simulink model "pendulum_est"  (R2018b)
settings: Solver=ode4  StartTime=0.0  StopTime=T  FixedStep=1e-3  RelTol=1e-3
model workspace (MAT data in the model file):
  pendulum_down1 : sldodialogs.data.SessionData (value not decoded)
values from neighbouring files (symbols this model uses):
  dtheta0 = mean(dtheta(n_start-5:n_start+5))    [mainSkript_odhadKyvadlaZvlast.m]    (also in mainSkript_pocitaniTVLQR_simplified.m = traj.dth_0; mainSkript_provedeniSimulaceSwingUp.m = [dtheta0 , stbVc])
  k_1 = params.k_1    [mainSkript_odhadKyvadlaZvlast.m]    (also in mainSkript_estimaceVozik.m = 1 / m; mainSkript_kyvadlaNajednouOdhad.m; mainSkript_modifikaceVozik.m = 0.695894224078)
  k_2 = params.k_2    [mainSkript_odhadKyvadlaZvlast.m]    (also in mainSkript_kyvadlaNajednouOdhad.m)
  theta0 = theta_cut(1)    [mainSkript_odhadKyvadlaZvlast.m]    (also in mainSkript_pocitaniTVLQR_simplified.m = traj.th_0; mainSkript_provedeniSimulaceSwingUp.m = [theta0 , stbVc])

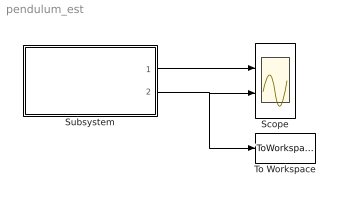
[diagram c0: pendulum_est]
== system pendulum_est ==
  Scope : Scope  NumInputPorts=2
  Subsystem : Subsystem
  To Workspace : ToWorkspace  VariableName=th_sim  SaveFormat=Structure With Time  SampleTime=-1
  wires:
  Subsystem/1(dtheta) -> Scope/1
  Subsystem/2(theta) -> To Workspace/1, Scope/2

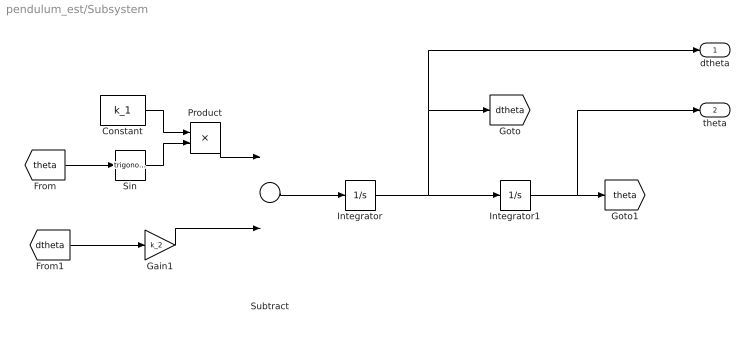
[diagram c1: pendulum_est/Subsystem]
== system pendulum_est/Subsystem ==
  Constant : Constant  Value=k_1
  Gain1 : Gain  Gain=k_2
  Integrator : Integrator  InitialCondition=dtheta0
  Integrator1 : Integrator  InitialCondition=theta0
  Product : Product
  Sin : Trigonometry
  Subtract : Sum  Inputs=+-
  dtheta : Outport
  theta : Outport  Port=2
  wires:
  Constant/1 -> Product/1
  Product/1 -> Subtract/1
  Gain1/1 -> Subtract/2
  Integrator/1 -> Integrator1/1, dtheta/1, [dtheta]
  [dtheta] -> Gain1/1
  Integrator1/1 -> theta/1, [theta]
  Subtract/1 -> Integrator/1
  Sin/1 -> Product/2
  [theta] -> Sin/1
